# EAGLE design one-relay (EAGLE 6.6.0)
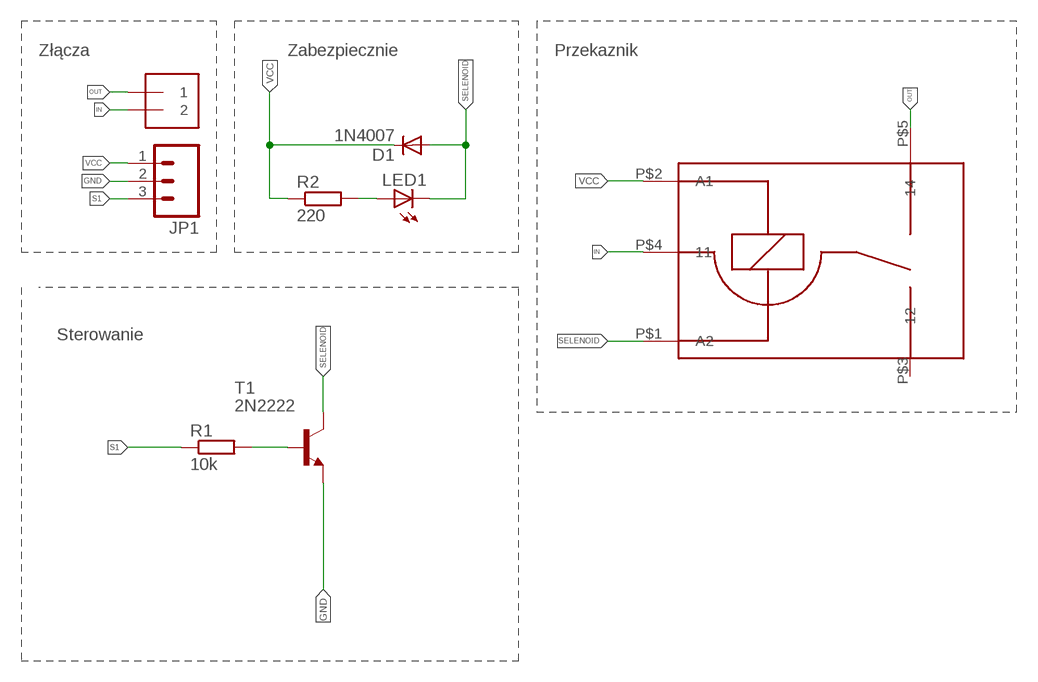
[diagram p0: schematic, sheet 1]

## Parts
D1  1N4007  1N4004  [DO41-10]
J1  1X2-3.5MM  [1X2-3.5MM]
JP1  M03SCREW  [SCREWTERMINAL-3.5MM-3]
LED1  LED3MM  [LED3MM]
R1  10k  R-EU_0204/7  [0204/7]
R2  220  R-EU_0204/7  [0204/7]
T1  2N2222  [TO92-EBC-OVAL]
U$1  RM96P  [RM96]

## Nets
GND: JP1.2 T1.E
IN: J1.2 U$1.P$4
N$2: LED1.A R2.2
N$4: R1.2 T1.B
OUT: J1.1 U$1.P$5
S1: JP1.3 R1.1
SELENOID: D1.A LED1.K(C) T1.C U$1.P$1(A2)
VCC: D1.C JP1.1 R2.1 U$1.P$2(A1)
Unconnected: U$1.P$3

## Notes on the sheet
- Złącza | Zabezpiecznie | Przekaznik
- Sterowanie

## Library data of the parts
D1 = adafruit:1N4004: DIODE
J1 = adafruit:1X2: 3.5mm Terminal block
JP1 = SparkFun-Connectors:M03: Header 3 Standard 3-pin 0.1" header. Use with straight break away headers (SKU : PRT-00116), right angle break away headers (PRT-00553), swiss pins (PRT-00743), machine pins (PRT-00117), and female headers (PRT-00115). Molex polarized connector foot print use with SKU : PRT-08232 with associated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
LED1 = led:LED: LED
R1 R2 = resistor:R-EU_: RESISTOR, European symbol
T1 = adafruit:2N2222: NPN TRANSISTOR Big oval pads
U$1 = nettigo:RM96P

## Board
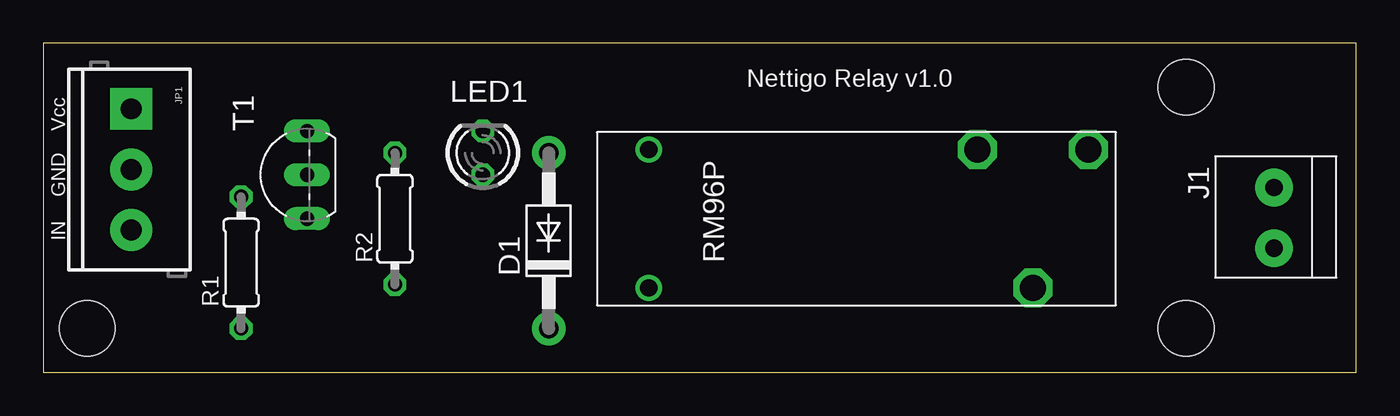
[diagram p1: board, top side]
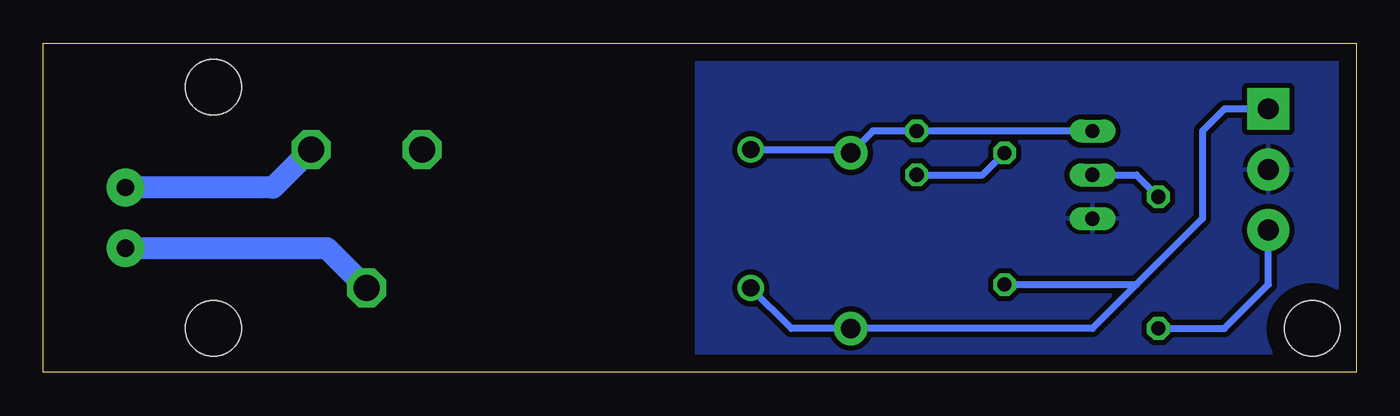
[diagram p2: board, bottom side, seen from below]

Size 75.87 x 19.04 mm. Coordinates in mm from the lower left corner, seen from the top.
Outline: 0,0 75.87,0 75.87,19.04 0,19.04 0,0
Copper layers (1*16): Top 0.035mm / dielectric 1.5mm / Bottom 0.035mm
Design rules "default": minimum track width 10mil, minimum drill 24mil, track to track 8mil, track to pad 8mil, pad to pad 8mil, via to via 8mil, smd to smd 8mil, copper to edge 40mil, drill to drill 8mil, minimum pad ring 10mil, minimum via ring 8mil, stop-mask expansion 4mil, vias tented up to drill 0mil, thermal gap 10mil
Holes 3.2 mm at 2.54,2.54 66.04,16.51 66.04,2.54

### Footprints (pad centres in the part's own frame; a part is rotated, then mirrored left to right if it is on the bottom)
DO41-10 = drill 1.118 pad 1.93: A 5.08,0; C -5.08,0
1X2-3.5MM = drill 1 pad 2.184: 1 1.8,0; 2 -1.7,0
SCREWTERMINAL-3.5MM-3 = drill 1.2 pad 2.413 square: 1 0,0 | drill 1.2 pad 2.413: 2 3.5,0; 3 7,0
LED3MM = drill 0.813 octagon: A -1.27,0; K 1.27,0
0204/7 = drill 0.813 octagon: 1 -3.81,0; 2 3.81,0
TO92-EBC-OVAL = drill 0.813 long: B 0,-1.27; C 2.54,-1.27; E -2.54,-1.27
RM96 = drill 1: P$1 -12,4; P$2 -12,-4 | drill 1.5 octagon: P$3 7,4; P$4 10.2,-4; P$5 13.4,4

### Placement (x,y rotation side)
D1  29.21,7.62 90 top
DRILEGEND  [DRILEGEND]  not placed on the board
J1  71.12,8.89 90 top
JP1  5.08,15.24 270 top
LED1  25.4,12.7 90 top
R1  11.43,6.35 90 top
R2  20.32,8.89 90 top
T1  13.97,11.43 90 top
U$1  46.99,8.89 0 top

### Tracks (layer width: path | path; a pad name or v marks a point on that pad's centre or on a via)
GND
  pour Bottom (isolate 0.305): 0,19.05 0,0 38.1,0 38.1,19.05
IN
  Bottom 1.27: J1.2 59.49,7.19 U$1.P$4
N$2
  Bottom 0.406: LED1.A 21.59,11.43 R2.2
N$4
  Bottom 0.406: T1.B 12.7,11.43 R1.2
OUT
  Bottom 1.27: U$1.P$5 62.59,10.69 J1.1
S1
  Bottom 0.406: R1.1 7.62,2.54 5.08,5.08 JP1.3
SELENOID
  Bottom 0.406: U$1.P$1 29.4,12.89 D1.A 27.94,13.97 LED1.K T1.C
VCC
  Bottom 0.406: JP1.1 7.62,15.24 8.89,13.97 8.89,8.89 12.7,5.08 | 12.7,5.08 15.24,2.54 D1.C 32.64,2.54 U$1.P$2 | R2.1 12.7,5.08

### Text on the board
tNames: Nettigo Relay v1.0 | Vcc | GND | IN
DrillLegend: LAYER-STACK
DrillLegend_01-16: 01-16
DrillLegend_01-20: 01-20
